DATA_BLOCK "Demo3"
VERSION : 0.1


  STRUCT
   str1 : STRING  [254 ] := '789 IJKLMNOP$R';	//write $$ to insert one single $; write $R to insert <CR> (0d hex)
  END_STRUCT ;
BEGIN
   str1 := '789 IJKLMNOP$R';
END_DATA_BLOCK

